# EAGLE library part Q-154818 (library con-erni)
Male Connector SMC-Q 12 contacts Type 7-13 - Low Profile Source: http://www.erni.com/DB/PDF-Drawing/SMC/154818.pdf
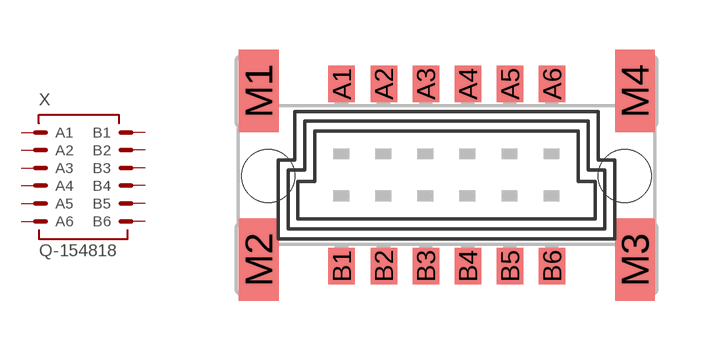
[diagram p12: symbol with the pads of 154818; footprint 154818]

Designator prefix X

## Q-154818 (OC_FARNELL: unknown; OC_NEWARK: unknown)  [154818]
A1  A1  pas
A2  A2  pas
A3  A3  pas
A4  A4  pas
A5  A5  pas
A6  A6  pas
B1  B1  pas
B2  B2  pas
B3  B3  pas
B4  B4  pas
B5  B5  pas
B6  B6  pas

## Footprint 154818 (pad centres in mm)
Male Connector SMC-Q 12 contacts Type 7-13 - Low Profile Source: http://www.erni.com/DB/PDF-Drawing/SMC/154818.pdf
smd 0.8 x 1.1: A1 -3.175,2.765; A2 -1.905,2.765; A3 -0.635,2.765; A4 0.635,2.765; A5 1.905,2.765; A6 3.175,2.765; B1 -3.175,-2.74; B2 -1.905,-2.74; B3 -0.635,-2.74; B4 0.635,-2.74; B5 1.905,-2.74; B6 3.175,-2.74
smd 1.2 x 2.5: M1 -5.68,2.55; M2 -5.68,-2.55; M3 5.68,-2.55; M4 5.68,2.55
